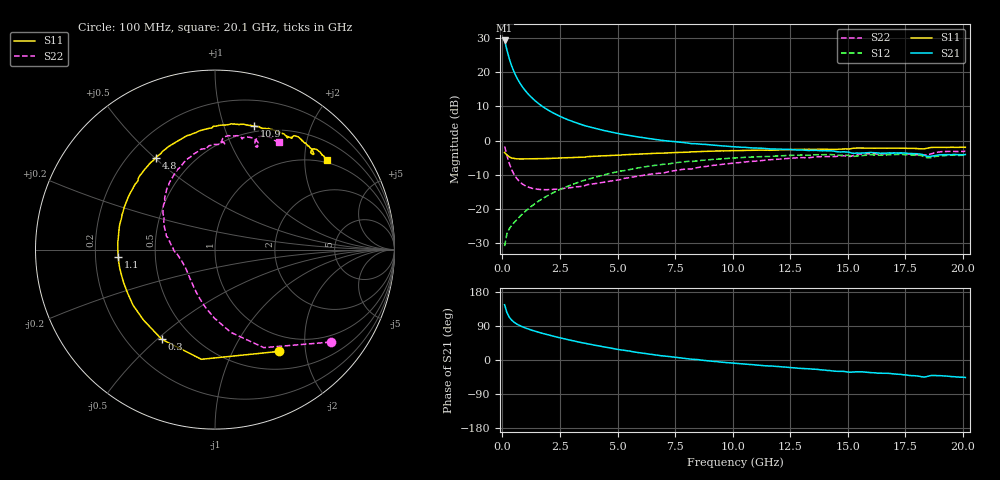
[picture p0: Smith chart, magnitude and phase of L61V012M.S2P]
!  Infineon Technologies AG
! BFR380L3 , PF131585-7, No.6, Th 09.10.01, soldered on pcb-board, measured with PP GSG850
!  Vce=1.0 V,  Ic=12.5 mA
! Common Emitter S-Parameters:  15. November 2001
#  GHz  S  MA  R  50
! f  S11  S21  S12  S22
! GHz  Mag  Ang  Mag  Ang  Mag  Ang  Mag  Ang
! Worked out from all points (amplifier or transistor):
!   201 points, 100 MHz to 20.1 GHz, reference 50 ohm
!   highest |S21| = 29.2 dB at 100 MHz (marker M1)
!   |S21| within 3 dB of that: start of sweep to 209.6 MHz
!   unconditionally stable (mu >= 1): 1.583 GHz to 4.964 GHz
!   at 3.4 GHz: K = 1.03, MAG = 7.3 dB, |S12| = -11.9 dB
!   at 10.1 GHz: K = 0.97, MSG = 1.6 dB, |S12| = -5.1 dB
!   at 20.1 GHz: K = 0.99, MSG = 0.1 dB, |S12| = -4.2 dB
!   S11 on the Smith chart (normalised r, x): 100 MHz: 0.75, -1.54; 300 MHz: 0.34, -0.52; 1.1 GHz: 0.30, -0.03; 4.8 GHz: 0.31, +0.50; 10.9 GHz: 0.44, +1.27; 20.1 GHz: 0.93, +2.56
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0.1  0.67 -57.8  28.91 145.9  0.02889 62.9  0.8246 -38.7
0.2  0.6159 -97.1  21.04 125.0  0.04381 52.7  0.6105 -63.5
0.3  0.5814 -120.7  15.81 113.2  0.05172 48.9  0.4692 -79.2
0.4  0.5593 -135.5  12.47 105.6  0.05769 48.2  0.3818 -90.5
0.5  0.5518 -145.8  10.24 100.1  0.06317 49.3  0.3262 -99.3
0.6  0.5437 -153.5  8.655 96.0  0.06871 50.5  0.2887 -106.6
0.7  0.5416 -159.8  7.503 92.5  0.07469 51.9  0.2627 -112.9
0.8  0.5402 -164.7  6.609 89.5  0.08085 53.2  0.2437 -118.3
0.9  0.5408 -168.9  5.909 86.9  0.08684 54.3  0.2295 -123.1
1.1  0.5404 -175.9  4.885 82.3  0.09959 55.9  0.2122 -131.4
1.3  0.5417 178.3  4.163 78.2  0.1126 57.1  0.2014 -138.0
1.5  0.5426 173.4  3.634 74.5  0.126 57.6  0.1959 -143.6
2  0.5493 163.0  2.775 66.1  0.1598 57.6  0.1927 -154.5
2.6  0.5603 152.6  2.185 57.2  0.2003 55.9  0.1995 -164.6
3.5  0.5746 139.0  1.686 45.1  0.2606 51.4  0.2162 -175.9
4.8  0.6097 122.8  1.319 30.4  0.3401 43.5  0.2604 168.7
6.8  0.6551 101.8  1.027 12.1  0.4445 29.9  0.3344 147.5
10.1  0.7163 77.3  0.8125 -8.7  0.5591 8.7  0.4725 119.4
10.9  0.7229 72.4  0.7824 -12.4  0.5775 3.9  0.4984 112.7
13.5  0.7469 59.9  0.7197 -24.3  0.6178 -11.4  0.5736 94.0
16.8  0.7783 47.7  0.6641 -35.4  0.6207 -26.7  0.6503 74.4
20.1  0.7992 38.6  0.6263 -46.1  0.6135 -40.0  0.6988 59.1
